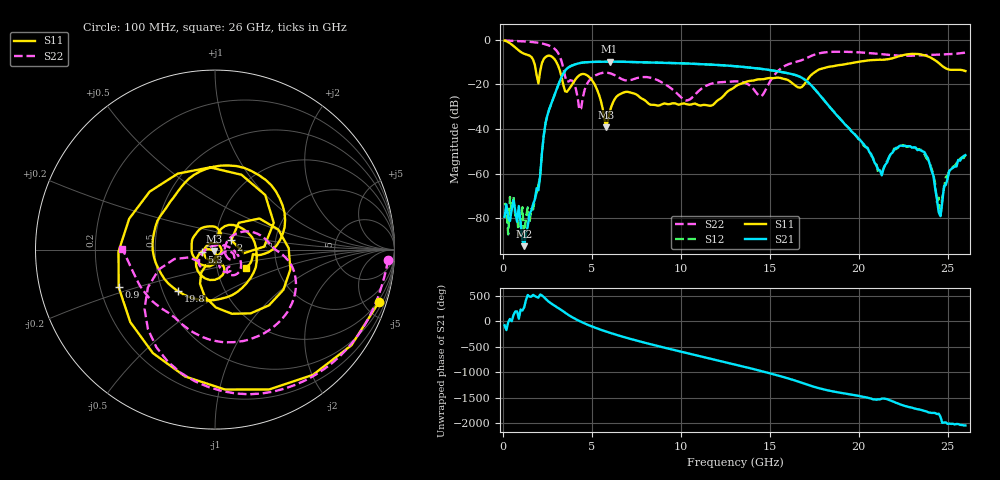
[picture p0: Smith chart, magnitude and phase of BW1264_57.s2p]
!Keysight Technologies,N5245B,MY57181159,A.13.60.06
!Date: Friday, December 18, 2020 23:55:04
!Correction: S11(Full 2 Port(1,2))
!S21(Full 2 Port(1,2))
!S12(Full 2 Port(1,2))
!S22(Full 2 Port(1,2))
!S2P File: Measurements: S11, S21, S12, S22:
# Hz S  dB  R 50
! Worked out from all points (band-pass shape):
!   260 points, 100 MHz to 26 GHz, reference 50 ohm
!   highest |S21| = -9.79 dB at 6 GHz (marker M1); lowest = -92.5 dB at 1.2 GHz (marker M2)
!   |S21| within 3 dB of the highest: 3.627 GHz to 14.27 GHz (10.65 GHz wide, 119 % of centre)
!   lowest |S11| = -39.3 dB at 5.8 GHz (marker M3), VSWR 1.02, Z = 49.3 - j0.815 ohm
!   |S11| at or under -10 dB: 1.748 GHz to 2.222 GHz (474.8 MHz wide, 23.9 % of centre); 3.011 GHz to 19.92 GHz (16.91 GHz wide, 147 % of centre); 24.44 GHz to end of sweep
!   |S22| runs from -31.4 to -0.3 dB; largest |S21 - S12| = 0.00058
!   S11 on the Smith chart (normalised r, x): 100 MHz: 0.86, -6.25; 900 MHz: 0.28, -0.17; 2 GHz: 1.19, +0.13; 5.3 GHz: 0.86, -0.02; 19.8 GHz: 0.60, -0.31; 26 GHz: 1.37, -0.30
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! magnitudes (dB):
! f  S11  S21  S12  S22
! 100 MHz  -0.4  -79.4  -73.1  -0.3
! 900 MHz  -4.8  -74.5  -87.8  -0.6
! 1.2 GHz  -6.3  -92.5  -89.3  -0.7
! 2 GHz  -19.6  -67.5  -65.1  -1.4
! 2.6 GHz  -7.1  -31.3  -31.3  -2.6
! 3.5 GHz  -23.1  -13.9  -13.9  -16.4
! 4.5 GHz  -15.3  -10.2  -10.2  -25.7
! 5.3 GHz  -22.4  -9.9  -9.9  -15.6
! 5.8 GHz  -39.3  -9.8  -9.8  -14.7
! 6 GHz  -32.6  -9.8  -9.8  -15.0
! 8.8 GHz  -29.4  -10.2  -10.2  -18.5
! 10.3 GHz  -28.8  -10.6  -10.6  -27.2
! 13.1 GHz  -20.8  -11.9  -11.9  -18.6
! 14.5 GHz  -17.7  -13.0  -13.0  -25.3
! 17.4 GHz  -15.3  -21.0  -21.0  -7.0
! 19.8 GHz  -10.2  -42.5  -42.5  -5.5
! 21.3 GHz  -9.0  -60.7  -59.7  -6.5
! 21.7 GHz  -8.6  -52.7  -53.0  -6.8
! 23.7 GHz  -6.9  -50.3  -51.3  -6.9
! 24.6 GHz  -11.1  -79.0  -79.0  -6.6
! 24.9 GHz  -12.8  -65.0  -61.5  -6.6
! 26 GHz  -14.0  -51.7  -51.7  -5.7
